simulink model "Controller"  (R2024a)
settings: Solver=odeN  StartTime=0.0  StopTime=1  FixedStep=Ts  MaxStep=10e-6  RelTol=1e-3  AbsTol=1e-4  EnableMultiTasking=on
PreLoadFcn:
  | TotemPole_PFCData;
StopFcn:
  | out.getSimulationMetadata.TimingInfo

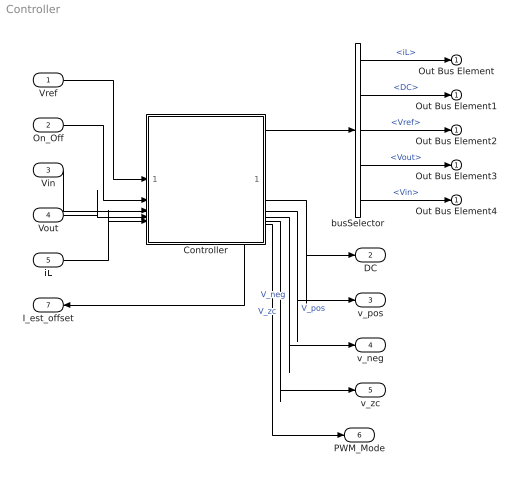
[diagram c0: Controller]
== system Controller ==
  Vref : Inport  OutDataTypeStr=single  PortDimensions=1  SampleTime=[0.01,0]
  On_Off : Inport  Port=2  OutDataTypeStr=double  PortDimensions=1  SampleTime=[0,1]
  Vin : Inport  Port=3  OutDataTypeStr=single  PortDimensions=1  SampleTime=[1.0000000000000001e-05,0]
  Vout : Inport  Port=4  OutDataTypeStr=single  PortDimensions=1  SampleTime=[1.0000000000000001e-05,0]
  iL : Inport  Port=5  OutDataTypeStr=single  PortDimensions=1  SampleTime=[1.0000000000000001e-05,0]
  Controller : Subsystem  TreatAsAtomicUnit=on  ReferencedSubsystem=Control
  busSelector : BusSelector  OutputSignals=iL,DC,Vref,Vout,Vin
  Out Bus Element{,1..4} (5 alike) : Outport
  DC : Outport  Port=2  OutDataTypeStr=single  PortDimensions=1  SampleTime=[1.0000000000000001e-05,0]
  v_pos : Outport  Port=3  OutDataTypeStr=uint16  PortDimensions=1  SampleTime=[1.0000000000000001e-05,0]
  v_neg : Outport  Port=4  OutDataTypeStr=uint16  PortDimensions=1  SampleTime=[1.0000000000000001e-05,0]
  v_zc : Outport  Port=5  OutDataTypeStr=uint16  PortDimensions=1  SampleTime=[1.0000000000000001e-05,0]
  PWM_Mode : Outport  Port=6  OutDataTypeStr=uint16  PortDimensions=1  SampleTime=[1.0000000000000001e-05,0]
  I_est_offset : Outport  Port=7  OutDataTypeStr=single  PortDimensions=1  SampleTime=[1.0000000000000001e-05,0]
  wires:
  Vref/1 -> Controller/1
  On_Off/1 -> Controller/2
  Vin/1 -> Controller/3
  Vout/1 -> Controller/4
  iL/1 -> Controller/5
  Controller/6 -> PWM_Mode/1
  Controller/7 -> I_est_offset/1
  Controller/1 -> busSelector/1
  Controller/5 -> v_zc/1  "V_zc"
  Controller/4 -> v_neg/1  "V_neg"
  Controller/3 -> v_pos/1  "V_pos"
  Controller/2 -> DC/1
  busSelector/4 -> Out Bus Element3/1  "<Vout>"
  busSelector/3 -> Out Bus Element2/1  "<Vref>"
  busSelector/2 -> Out Bus Element1/1  "<DC>"
  busSelector/1 -> Out Bus Element/1  "<iL>"
  busSelector/5 -> Out Bus Element4/1  "<Vin>"
